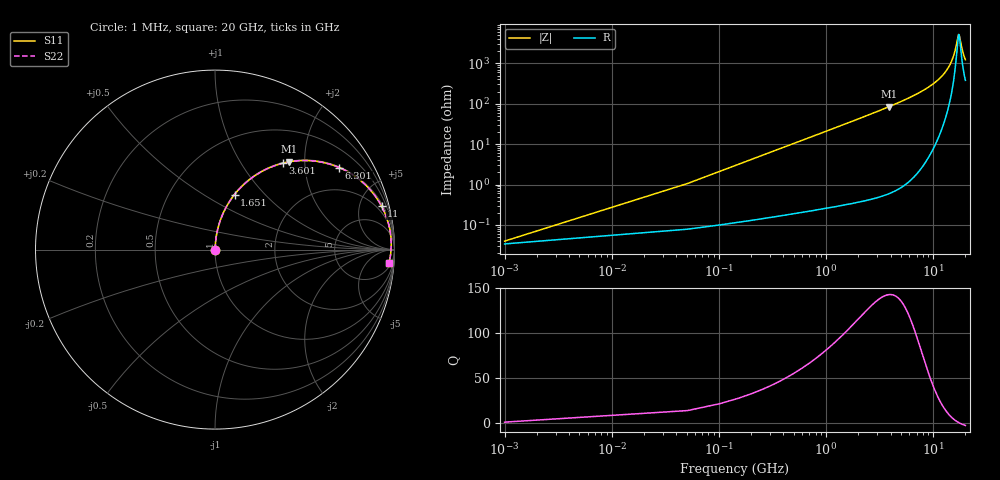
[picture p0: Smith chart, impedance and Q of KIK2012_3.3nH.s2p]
!version-2
!date-01.2022
!Series
# MHz S RI R 50
!Freq ReS11 ImS11 ReS21 ImS21 ReS12 ImS12 ReS22 ImS22
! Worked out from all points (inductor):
!   401 points, 1 MHz to 20 GHz, reference 50 ohm
!   read as one part in series: L = 3.3 nH near 101 MHz
!   highest Q = 143 at 3.851 GHz (marker M1), where L = 3.47 nH
!   self-resonance near 17.39 GHz
!   S11 on the Smith chart (normalised r, x): 1 MHz: 1.00, +0.00; 1.651 GHz: 1.01, +0.69; 3.601 GHz: 1.01, +1.56; 6.301 GHz: 1.03, +3.01; 11 GHz: 1.26, +7.61; 20 GHz: 9, -23
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1  0.000338 0.000207  0.9997 -0.000207  0.9997 -0.000207  0.000338 0.000207
151  0.00213 0.0312  0.9979 -0.0312  0.9979 -0.0312  0.00213 0.0312
251  0.0041 0.0518  0.9959 -0.0518  0.9959 -0.0518  0.0041 0.0518
351  0.00687 0.0722  0.9931 -0.0722  0.9931 -0.0722  0.00687 0.0722
551  0.0148 0.1124  0.9852 -0.1124  0.9852 -0.1124  0.0148 0.1124
851  0.0325 0.1707  0.9675 -0.1707  0.9675 -0.1707  0.0325 0.1707
1651  0.1089 0.3068  0.8911 -0.3068  0.8911 -0.3068  0.1089 0.3068
3351  0.3436 0.4713  0.6564 -0.4713  0.6564 -0.4713  0.3436 0.4713
3601  0.3793 0.4817  0.6207 -0.4817  0.6207 -0.4817  0.3793 0.4817
3851  0.4142 0.4891  0.5858 -0.4891  0.5858 -0.4891  0.4142 0.4891
6301  0.6921 0.4572  0.3079 -0.4572  0.3079 -0.4572  0.6921 0.4572
6701  0.7253 0.4416  0.2747 -0.4416  0.2747 -0.4416  0.7253 0.4416
10001  0.9002 0.2878  0.0998 -0.2878  0.0998 -0.2878  0.9002 0.2878
11001  0.9283 0.2415  0.0717 -0.2415  0.0717 -0.2415  0.9283 0.2415
13351  0.9674 0.1414  0.0326 -0.1414  0.0326 -0.1414  0.9674 0.1414
15301  0.9802 0.0684  0.0198 -0.0684  0.0198 -0.0684  0.9802 0.0684
16051  0.9818 0.0428  0.0182 -0.0428  0.0182 -0.0428  0.9818 0.0428
16701  0.9819 0.0215  0.0181 -0.0215  0.0181 -0.0215  0.9819 0.0215
17151  0.9815 0.00732  0.0185 -0.00732  0.0185 -0.00732  0.9815 0.00732
17451  0.9809 -0.00191  0.0191 0.00191  0.0191 0.00191  0.9809 -0.00191
18801  0.9764 -0.0412  0.0236 0.0412  0.0236 0.0412  0.9764 -0.0412
20000  0.97 -0.0732  0.03 0.0732  0.03 0.0732  0.97 -0.0732
